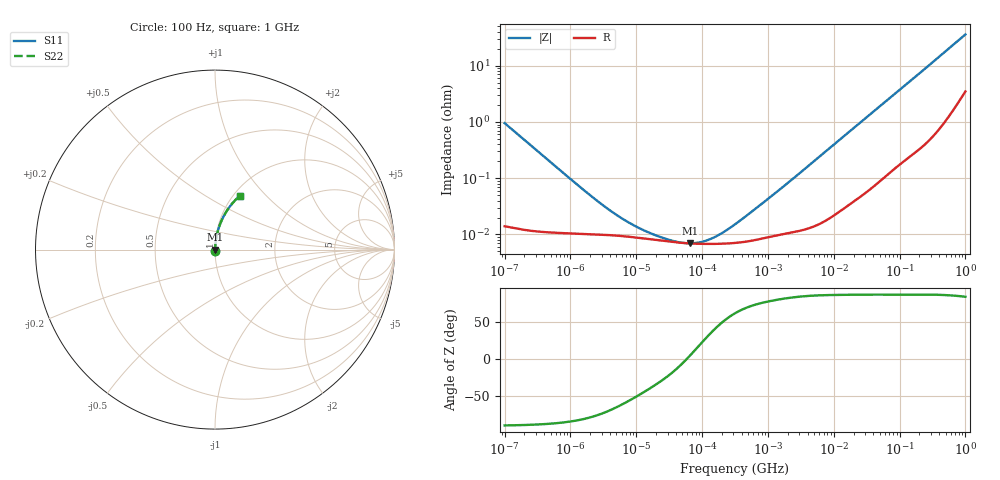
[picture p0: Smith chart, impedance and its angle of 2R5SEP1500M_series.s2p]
!  *** S-Parameter ***
!  Copyright (C) Panasonic Industry Corporation
!  Conductive Polymer Aluminum Soild Capacitor (OS-CON)
!  Parts No. 2R5SEP1500M
!  Connection Mode : Series
!  1  o---||---o  2
!  GND o--------o GND
!  Conditions : Temperature = 20 degC  DC Bias = 0 V
! Frequency Range : 100Hz  -  1GHz  [ 401 Steps ]
# Hz S RI R 50
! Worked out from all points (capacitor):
!   401 points, 100 Hz to 1 GHz, reference 50 ohm
!   read as one part in series: C = 1.66 mF near 108.4 Hz
!   lowest |Z| = 6.96 mohm at 65.69 kHz (marker M1)
!   series resonance near 57.8 kHz, so ESL is about 4.6 nH
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100  0.000231 -0.00955  0.9998 0.00955  0.9998 0.00955  0.000231 -0.00955
108.3927  0.000215 -0.00881  0.9998 0.00881  0.9998 0.00881  0.000215 -0.00881
1487.647  0.000103 -0.000651  0.9999 0.000651  0.9999 0.000651  0.000103 -0.000651
3467.369  9.82e-05 -0.000285  0.9999 0.000285  0.9999 0.000285  9.82e-05 -0.000285
6878.599  9.23e-05 -0.00015  0.9999 0.00015  0.9999 0.00015  9.23e-05 -0.00015
10715.19  8.72e-05 -9.94e-05  0.9999 9.94e-05  0.9999 9.94e-05  8.72e-05 -9.94e-05
16691.68  8.19e-05 -6.47e-05  0.9999 6.47e-05  0.9999 6.47e-05  8.19e-05 -6.47e-05
18836.49  8.04e-05 -5.7e-05  0.9999 5.7e-05  0.9999 5.7e-05  8.04e-05 -5.7e-05
22130.95  7.85e-05 -4.76e-05  0.9999 4.76e-05  0.9999 4.76e-05  7.85e-05 -4.76e-05
65690.11  6.93e-05 6.31e-06  0.9999 -6.31e-06  0.9999 -6.31e-06  6.93e-05 6.31e-06
179887.1  6.82e-05 7.07e-05  0.9999 -7.07e-05  0.9999 -7.07e-05  6.82e-05 7.07e-05
211348.9  6.86e-05 8.58e-05  0.9999 -8.58e-05  0.9999 -8.58e-05  6.86e-05 8.58e-05
316227.8  7.06e-05 0.000134  0.9999 -0.000134  0.9999 -0.000134  7.06e-05 0.000134
1244515  9.43e-05 0.000516  0.9999 -0.000516  0.9999 -0.000516  9.43e-05 0.000516
4704354  0.000139 0.00188  0.9999 -0.00188  0.9999 -0.00188  0.000139 0.00188
2.357762e7  0.000522 0.0091  0.9995 -0.0091  0.9995 -0.0091  0.000522 0.0091
6.99842e7  0.00192 0.0262  0.9981 -0.0262  0.9981 -0.0262  0.00192 0.0262
1.566751e8  0.00587 0.057  0.9941 -0.057  0.9941 -0.057  0.00587 0.057
2.985383e8  0.0165 0.106  0.9835 -0.106  0.9835 -0.106  0.0165 0.106
5.688529e8  0.0517 0.1922  0.9483 -0.1922  0.9483 -0.1922  0.0517 0.1922
9.225714e8  0.1202 0.2829  0.8798 -0.2829  0.8798 -0.2829  0.1202 0.2829
1e9  0.1373 0.2989  0.8627 -0.2989  0.8627 -0.2989  0.1373 0.2989
